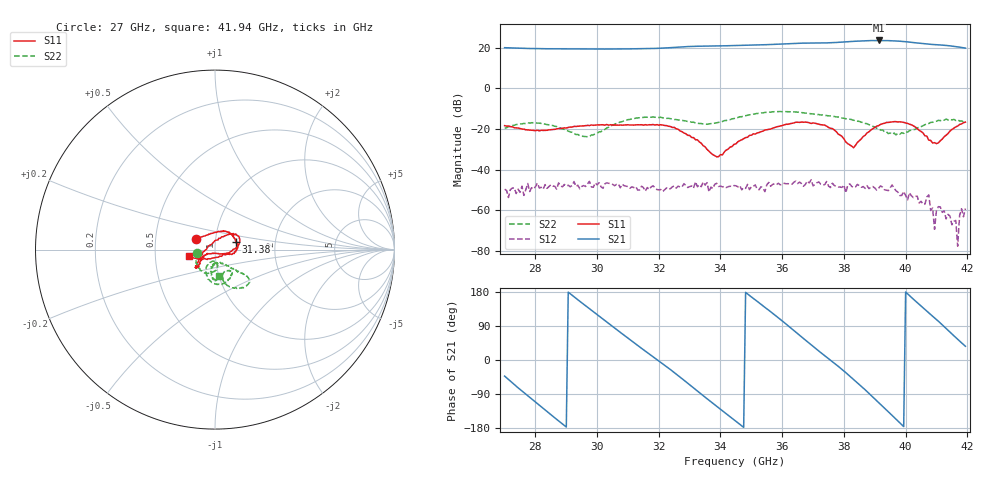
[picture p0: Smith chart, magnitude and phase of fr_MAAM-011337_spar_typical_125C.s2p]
! Created Thu Jan 25 15:58:37 2024
# hz S db R 50
! 2 Port Network Data from SP1.SP block
! freq  dbS11  angS11  dbS21  angS21  dbS12  angS12  dbS22  angS22
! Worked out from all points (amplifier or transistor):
!   240 points, 27 GHz to 41.94 GHz, reference 50 ohm
!   highest |S21| = 23.5 dB at 39.13 GHz (marker M1)
!   |S21| within 3 dB of that: 32.95 GHz to 41.62 GHz (8.677 GHz wide, 23.3 % of centre)
!   unconditionally stable (mu >= 1): start of sweep to end of sweep
!   at 29.5 GHz: K = 13.73, MAG = 19.3 dB, |S12| = -48.2 dB
!   at 34.5 GHz: K = 10.66, MAG = 21.2 dB, |S12| = -47.9 dB
!   at 41.94 GHz: K = 44.40, MAG = 19.9 dB, |S12| = -59.1 dB
!   S11 on the Smith chart (normalised r, x): 27 GHz: 0.81, +0.10; 31.38 GHz: 1.26, +0.11; 41.94 GHz: 0.75, -0.06
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2.70046e10  -18.36 149.9  19.92 -42.5  -49.60 -93.2  -19.62 -170.7
2.806689e10  -20.60 111.9  19.47 -115.3  -46.59 -104.2  -17.12 -110.9
2.881674e10  -19.74 77.6  19.32 -164.7  -47.99 -145.9  -19.47 -83.5
2.95041e10  -18.52 58.0  19.25 151.0  -48.18 -153.0  -23.53 -89.3
3.044141e10  -17.90 37.9  19.26 92.2  -46.90 162.2  -18.56 -115.0
3.137872e10  -17.98 20.2  19.39 34.7  -49.98 152.1  -14.48 -91.3
3.20036e10  -18.11 7.4  19.62 -2.8  -49.90 131.5  -14.38 -72.5
3.269096e10  -20.92 -15.4  20.27 -44.8  -48.46 117.4  -15.60 -54.6
3.331584e10  -26.32 -29.5  20.64 -86.0  -47.38 103.9  -17.33 -59.4
3.45031e10  -27.26 -147.6  21.00 -161.8  -47.89 78.9  -14.42 -74.6
3.519046e10  -21.94 -148.5  21.24 154.8  -49.56 50.6  -12.37 -63.4
3.60028e10  -18.32 -137.4  21.78 103.1  -47.23 34.5  -11.51 -47.7
3.644021e10  -16.69 -134.6  22.08 73.8  -45.59 25.5  -11.66 -42.4
3.70026e10  -17.03 -140.1  22.21 36.0  -47.94 -4.5  -12.63 -39.5
3.806489e10  -26.41 178.9  22.82 -33.5  -51.37 -30.4  -14.97 -42.7
3.862728e10  -23.65 71.9  23.25 -74.1  -48.27 -45.9  -16.85 -48.6
3.912718e10  -18.35 45.2  23.47 -112.2  -49.06 -73.7  -19.88 -57.2
3.95021e10  -16.65 32.6  23.35 -141.5  -48.87 -66.0  -21.93 -71.6
4.006449e10  -17.25 12.1  22.77 174.6  -54.82 -96.3  -21.57 -99.3
4.081434e10  -25.61 -46.1  21.59 120.0  -60.02 -147.2  -16.75 -97.8
4.131424e10  -23.05 -128.2  21.02 83.2  -64.15 31.5  -15.14 -91.2
4.193911e10  -16.64 -165.4  19.72 36.3  -59.07 -41.3  -16.61 -81.9
